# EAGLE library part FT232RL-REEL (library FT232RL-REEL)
USB/Serial IC UART SSOP-28 FTDI Chip FT232RL-REEL, USB Controller, 3MBd, USB 2.0, 1.8 5.25 V, 28-Pin SSOP Source: Datasheet
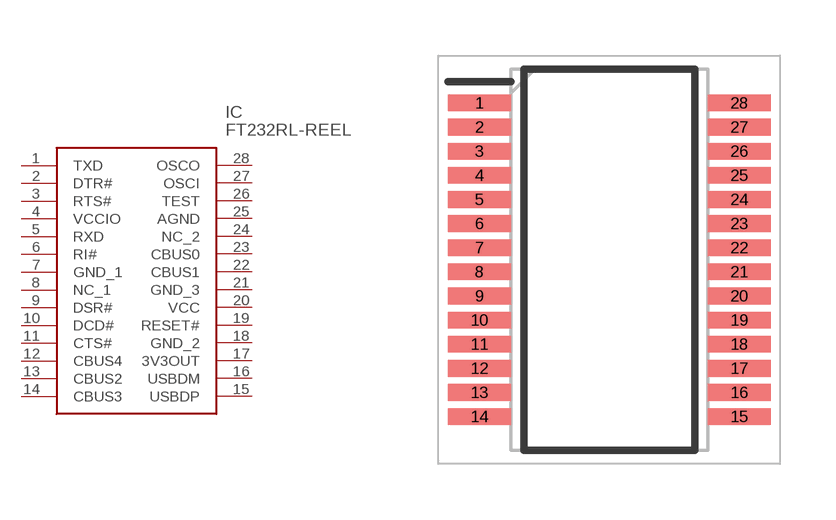
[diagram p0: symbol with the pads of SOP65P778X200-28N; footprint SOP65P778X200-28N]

Designator prefix IC

## FT232RL-REEL (Description: USB/Serial IC UART SSOP-28 FTDI Chip FT232RL-REEL, USB Controller, 3MBd, USB 2.0, 1.8 5.25 V, 28-Pin SSOP; Height: 2mm; Manufacturer_Name: FTDI Chip; Manufacturer_Part_Number: FT232RL-REEL; Mouser_Part_Number: 895-FT232RL; Mouser_Price-Stock: https://www.mouser.co.uk/ProductDetail/FTDI/FT232RL-REEL?qs=D1%2FPMqvA103RC6OU6bKtoA%3D%3D)  [SOP65P778X200-28N]
1  TXD
2  DTR#
3  RTS#
4  VCCIO
5  RXD
6  RI#
7  GND_1
8  NC_1
9  DSR#
10  DCD#
11  CTS#
12  CBUS4
13  CBUS2
14  CBUS3
15  USBDP
16  USBDM
17  3V3OUT
18  GND_2
19  RESET#
20  VCC
21  GND_3
22  CBUS1
23  CBUS0
24  NC_2
25  AGND
26  TEST
27  OSCI
28  OSCO

## Footprint SOP65P778X200-28N (pad centres in mm)
SSOP-28 1
smd 1.7 x 0.45: 1 -3.5,4.225; 2 -3.5,3.575; 3 -3.5,2.925; 4 -3.5,2.275; 5 -3.5,1.625; 6 -3.5,0.975; 7 -3.5,0.325; 8 -3.5,-0.325; 9 -3.5,-0.975; 10 -3.5,-1.625; 11 -3.5,-2.275; 12 -3.5,-2.925; 13 -3.5,-3.575; 14 -3.5,-4.225; 15 3.5,-4.225; 16 3.5,-3.575; 17 3.5,-2.925; 18 3.5,-2.275; 19 3.5,-1.625; 20 3.5,-0.975; 21 3.5,-0.325; 22 3.5,0.325; 23 3.5,0.975; 24 3.5,1.625; 25 3.5,2.275; 26 3.5,2.925; 27 3.5,3.575; 28 3.5,4.225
